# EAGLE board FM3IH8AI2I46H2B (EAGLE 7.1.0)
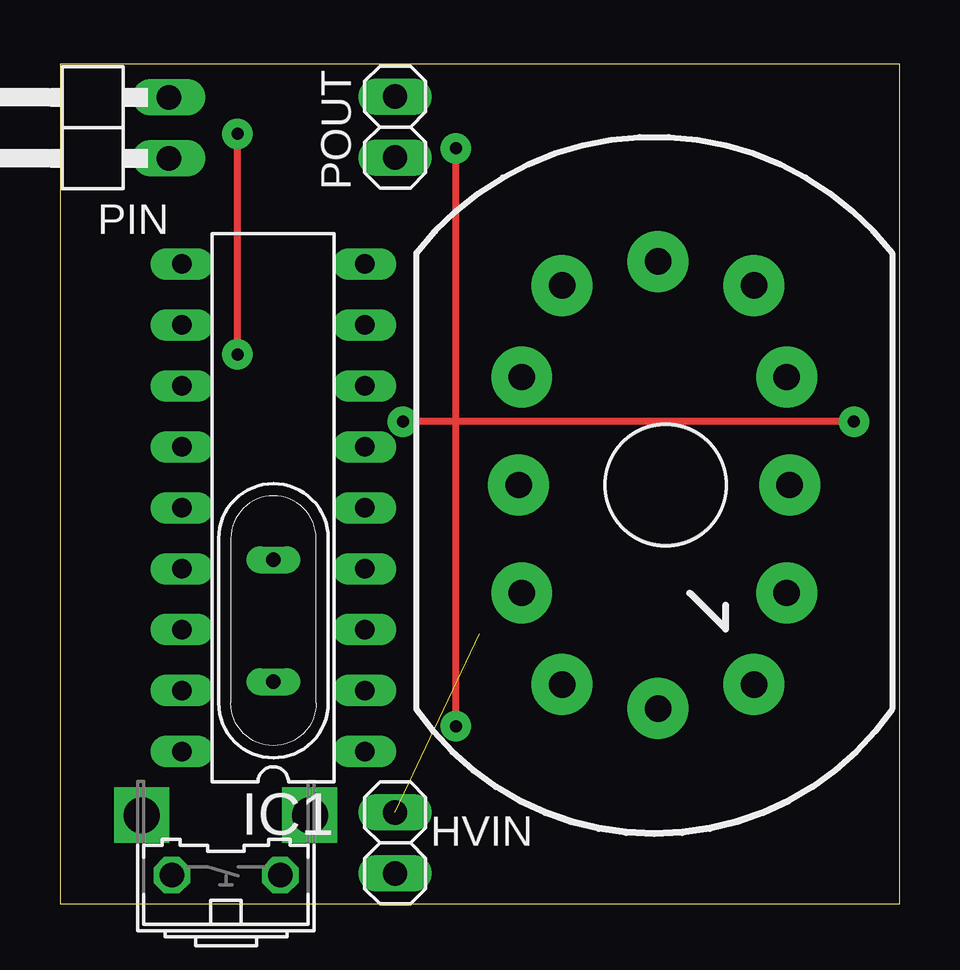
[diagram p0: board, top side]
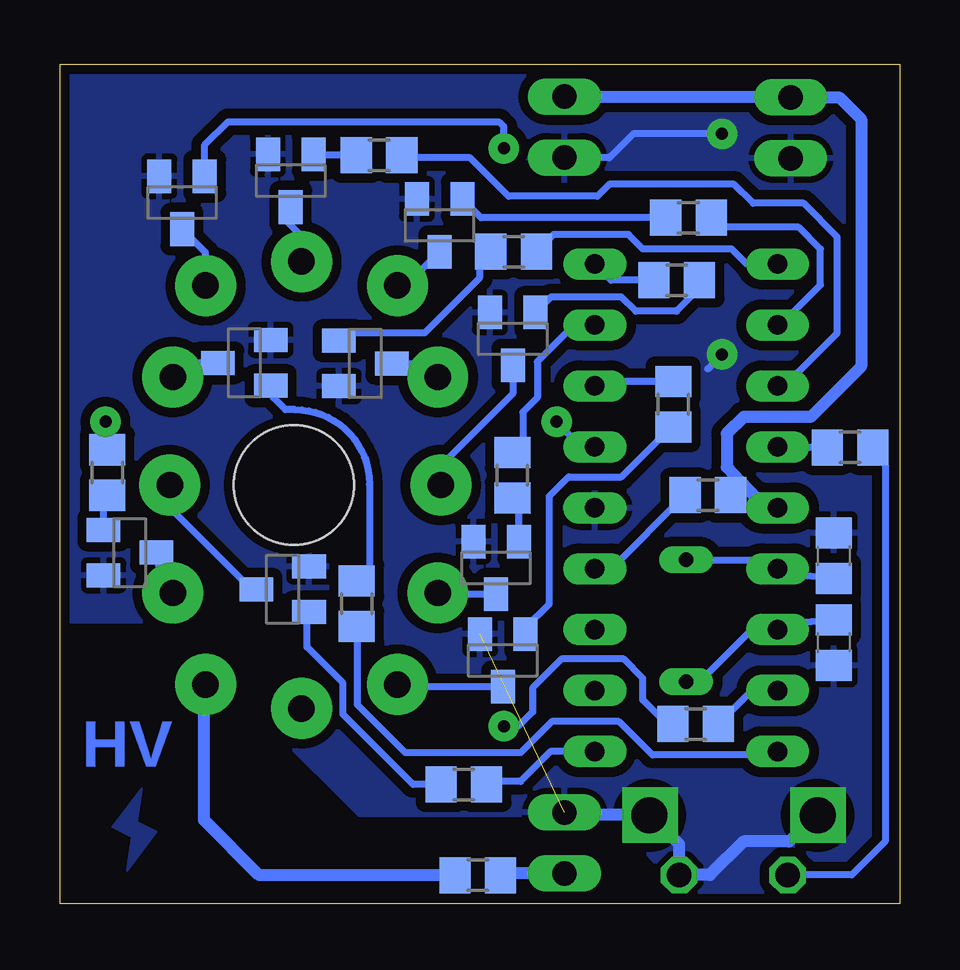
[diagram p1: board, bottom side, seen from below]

Size 35 x 35 mm. Coordinates in mm from the lower left corner, seen from the top.
Outline: 0,0 35,0 35,35 0,35 0,0
Copper layers (1*16): Top 0.035mm / dielectric 1.5mm / Bottom 0.035mm
Design rules "default *": minimum track width 0.2mm, minimum drill 0.4mm, track to track 0.25mm, track to pad 0.2mm, pad to pad 0.2mm, via to via 0.2mm, smd to smd 0.1mm, copper to edge 0.2mm, drill to drill 8mil, minimum pad ring 10mil, minimum via ring 8mil, stop-mask expansion 4mil, vias tented up to drill 0mil, thermal gap 10mil

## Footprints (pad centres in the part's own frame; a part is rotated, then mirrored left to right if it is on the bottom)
C0805 = smd 1.3 x 1.5: 1 -0.95,0; 2 0.95,0
1X02 = drill 1.016 long: 1 -1.27,0; 2 1.27,0
DIL18 = drill 0.813 long: 1 -10.16,-3.81; 2 -7.62,-3.81; 3 -5.08,-3.81; 4 -2.54,-3.81; 5 0,-3.81; 6 2.54,-3.81; 7 5.08,-3.81; 8 7.62,-3.81; 9 10.16,-3.81; 10 10.16,3.81; 11 7.62,3.81; 12 5.08,3.81; 13 2.54,3.81; 14 0,3.81; 15 -2.54,3.81; 16 -5.08,3.81; 17 -7.62,3.81; 18 -10.16,3.81
IN-12 = drill 1.1 pad 2.54: 0 5.048,-4.5; 1 -4.317,-8.318; 2 -6,-4.5; 3 -6.127,0; 4 -6,4.5; 5 -4.317,8.318; 6 -0.318,9.318; 7 3.683,8.318; 8 5.048,4.5; 9 5.175,0; A 3.683,-8.318; LHDP -0.318,-9.318 | hole 5: 0,0
1X02/90 = drill 1.016 long: 1 -1.27,-3.81; 2 1.27,-3.81
QS = drill 0.61 long: 1 -2.54,0; 2 2.54,0
R0805 = smd 1.3 x 1.5: 1 -0.95,0; 2 0.95,0
B3F-31XX = drill 1.016 octagon: 1 -2.261,-1.245; 2 2.261,-1.245 | drill 1.499 pad 2.159: 3 -3.505,1.245; 4 3.505,1.245
SOT23-BEC = smd 1 x 1.4: B -0.95,-1.1; C 0,1.1; E 0.95,-1.1

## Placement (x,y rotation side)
C1  22p  [C0805]  2.74,10.89 90 bottom
C2  22p  [C0805]  2.74,14.51 270 bottom
HVIN  [1X02]  13.97,2.54 270 top
IC1  PIC16F84AP  [DIL18]  8.89,16.51 90 top
N1  IN-12A  [IN-12]  25.25,17.46 0 top
PIN  [1X02/90]  0.73,32.35 90 top
POUT  [1X02]  13.97,32.38 90 top
Q1  [QS]  8.9,11.8 270 top
R1  100k  [R0805]  17.58,1.19 0 bottom
R2  1k  [R0805]  7.99,17.04 180 bottom
R3  470R  [R0805]  2.06,19.03 0 bottom
R5  [R0805]  9.43,20.82 270 bottom
R6  [R0805]  16.14,17.87 270 bottom
R7  [R0805]  9.29,26 0 bottom
R8  [R0805]  16.09,27.18 180 bottom
R9  [R0805]  8.8,28.6 180 bottom
R10  [R0805]  21.7,31.2 180 bottom
R11  [R0805]  8.5,7.5 180 bottom
R12  [R0805]  22.63,12.51 90 bottom
R13  [R0805]  18.16,4.98 180 bottom
R14  [R0805]  33.02,17.98 270 bottom
S1  [B3F-31XX]  6.92,2.44 0 top
T1  [SOT23-BEC]  16.54,10.15 180 bottom
T2  [SOT23-BEC]  16.82,14 180 bottom
T3  [SOT23-BEC]  16.12,23.55 180 bottom
T4  [SOT23-BEC]  22.27,22.53 270 bottom
T5  [SOT23-BEC]  19.18,28.29 180 bottom
T6  [SOT23-BEC]  25.38,30.14 180 bottom
T7  [SOT23-BEC]  29.91,29.23 180 bottom
T8  [SOT23-BEC]  27.32,22.55 90 bottom
T9  [SOT23-BEC]  25.71,13.12 90 bottom
T10  [SOT23-BEC]  32.09,14.64 270 bottom

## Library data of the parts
C1 C2 R1-R3 R5-R14 = rcl
HVIN PIN POUT = pinhead
IC1 = microchip; MF: MICROCHIP; MPN: PIC16F84A-04I/P; OC_FARNELL: 9760865; OC_NEWARK: 69K7635
N1 = russian-nixies
Q1 = special
S1 = switch-omron; MPN: B3F-3100; OC_FARNELL: 959704; OC_NEWARK: 36M3582
T1-T10 = transistor

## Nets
+5V: IC1.14 PIN.2 POUT.2 R2.1
GND: C1.1 C2.1 HVIN.1 IC1.5 PIN.1 POUT.1 S1.2 T1.E T2.E T3.E T4.E T5.E T6.E T7.E T8.E T9.E T10.E
N$1: N1.0 T10.C
N$2: N1.9 T9.C
N$3: N1.8 T8.C
N$4: N1.7 T7.C
N$5: N1.6 T6.C
N$6: N1.5 T5.C
N$7: N1.1 T1.C
N$8: N1.2 T2.C
N$9: N1.3 T3.C
N$10: N1.4 T4.C
N$11: C1.2 IC1.16 Q1.2
N$12: IC1.4 R2.2
N$13: C2.2 IC1.15 Q1.1
N$14: IC1.13 R3.1
N$15: R3.2 S1.1
N$16: IC1.6 R14.1
N$17: IC1.7 R5.1
N$18: R5.2 T1.B
N$19: R6.2 T2.B
N$20: R7.2 T3.B
N$21: IC1.8 R6.1
N$22: N1.A R1.1
N$23: IC1.9 R7.1
N$24: IC1.10 R8.1
N$25: IC1.11 R9.1
N$26: IC1.12 R10.1
N$27: IC1.17 R11.1
N$28: IC1.18 R12.1
N$29: IC1.1 R13.1
N$32: R8.2 T4.B
N$33: R9.2 T5.B
N$34: R10.2 T6.B
N$35: R11.2 T7.B
N$36: R12.2 T8.B
N$37: R13.2 T9.B
N$38: R14.2 T10.B
V+: HVIN.2 R1.2

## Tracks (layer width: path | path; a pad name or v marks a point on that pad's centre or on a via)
+5V
  Bottom 0.3: IC1.14 5.6,16.51 | R2.1 7.44,16.83 6.65,17.62
  Bottom 0.5: POUT.2 13.94,33.62 PIN.2 2.52,33.62 1.6,32.7 1.6,22.4 3.7,20.3 6.5,20.3 7.2,19.6 7.2,18.21 6.65,17.62 5.6,16.51
GND  (via drill 0.5 pad 1.27, 1 pad 2.3)  (1 unrouted)
  Top 0.3: v7.4,22.9 v7.4,32.1
  Bottom 0.3: 8,22.3 v7.4,22.9 | v7.4,32.1 11.1,32.1 12.1,31.1 13.96,31.1 POUT.1
  Bottom 0.5: v3.4,3.7 3.5,3.7 4.6,2.6 6.5,2.6 7.9,1.2 S1.2 9.18,2.48 v10.4,3.7 13.86,3.7 HVIN.1
  pour Bottom (isolate 0.4): 0.3,0.3 8.7,0.3 12.1,3.7 22.5,3.7 26.1,7.3 26.1,10.1 27.8,11.8 34.7,11.8 34.7,34.7 0.3,34.7
N$1
  Bottom 0.3: T10.C 30.89,14.05 N1.0
N$2
  Bottom 0.3: T9.C 26.82,12.91 30.3,16.4 30.3,17.34 N1.9
N$3
  Bottom 0.3: T8.C 29.7,22.55 N1.8
N$4
  Bottom 0.3: N1.7 28.93,27.15 T7.C
N$5
  Bottom 0.3: N1.6 24.93,27.83 25.6,28.5 25.6,28.82 T6.C
N$6
  Bottom 0.3: N1.5 20.58,25.78 T5.C
N$7
  Bottom 0.3: T1.C 20.84,9.05 N1.1
N$8
  Bottom 0.3: T2.C 19.19,12.9 N1.2
N$9
  Bottom 0.3: T3.C 16.12,21.27 19.1,18.3 19.1,17.48 N1.3
N$10
  Bottom 0.3: T4.C 19.82,22.53 N1.4
N$11
  Bottom 0.3: C1.2 4.87,11.64 IC1.16 5.11,11.4 6.2,11.4 8.34,9.26 Q1.2
N$12
  Bottom 0.3: IC1.4 12.01,13.97 R2.2
N$13
  Bottom 0.3: C2.2 4.87,13.76 IC1.15 5.45,14.34 Q1.1
N$14
  Bottom 0.3: R3.1 5.06,19.03 IC1.13
N$15
  Bottom 0.3: R3.2 1.11,18.81 0.6,18.3 0.6,2.6 2,1.2 S1.1
N$16  (via drill 0.5 pad 1.27)
  Top 0.3: v33.1,20.1 v14.3,20.1
  Bottom 0.3: v14.3,20.1 13.25,19 IC1.6 | v33.1,20.1 33.1,19.61 R14.1
N$17
  Bottom 0.3: R5.1 12.38,21.77 IC1.7
N$18
  Bottom 0.3: T1.B 15.59,11.51 14.6,12.5 14.6,17 13.8,17.8 11.6,17.8 10.1,19.3 9.4,19.9 R5.2
N$19
  Bottom 0.3: T2.B 15.87,17.25 R6.2
N$20
  Bottom 0.3: R7.2 8.34,25.66 9.3,24.7 11,24.7 11.6,25.3 14.53,25.3 T3.B
N$21
  Bottom 0.3: IC1.8 13.57,24.13 15.1,22.6 15.1,21.1 15.7,20.5 15.7,19.26 R6.1
N$22
  Bottom 0.5: R1.1 26.69,1.19 29,3.5 29,9.11 N1.A
N$23
  Bottom 0.3: R7.1 12.03,26 IC1.9
N$24
  Bottom 0.3: IC1.10 6.37,26.67 7,27.3 10.7,27.3 11.3,27.9 14.42,27.9 R8.1
N$25
  Bottom 0.3: IC1.11 4.97,24.13 3.3,25.8 3.3,27.3 4.2,28.2 7.45,28.2 R9.1
N$26
  Bottom 0.3: IC1.12 4.81,21.59 2.6,23.8 2.6,27.8 4,29.2 6.1,29.2 6.9,30 12.1,30 12.6,29.5 16.3,29.5 17.9,31.1 20.65,31.1 R10.1
N$27
  Bottom 0.3: IC1.17 6.16,8.89 R11.1
N$28
  Bottom 0.3: IC1.18 6.05,6.35 6.2,6.2 10.3,6.2 11.7,7.6 14.5,7.6 15.8,6.3 20.6,6.3 22.6,8.3 22.6,11.39 R12.1
N$29
  Bottom 0.3: IC1.1 14.55,6.35 15.8,5.1 17.09,5.1 R13.1
N$30
  pour Bottom: 31.6,4.8 31.8,3.4 31,3 32.2,1.4 32,2.8 32.8,3.2
N$32
  Bottom 0.3: R8.2 17.52,26.58 17.52,26.08 19.8,23.8 23.05,23.8 T4.B
N$33
  Bottom 0.3: R9.2 17.44,28.6 T5.B
N$34
  Bottom 0.3: R10.2 24.38,31.2 T6.B
N$35  (via drill 0.5 pad 1.27)
  Top 0.3: v16.5,7.4 v16.5,31.5
  Bottom 0.3: R11.2 9.7,7.5 10.7,8.5 10.7,9.4 11.5,10.2 14.1,10.2 15.3,9 15.3,8 15.9,7.4 v16.5,7.4 | v16.5,31.5 16.5,32.4 16.7,32.6 28,32.6 28.96,31.64 T7.B
N$36
  Bottom 0.3: R12.2 22.1,13.89 22.1,17.5 arc-90 25.2,20.6 25.6,20.6 26.1,21.1 26.1,21.59 T8.B
N$37
  Bottom 0.3: R13.2 20.28,4.98 23.2,7.9 23.2,9.2 24.7,10.7 24.7,12.08 T9.B
N$38
  Bottom 0.3: T10.B 33.19,16.47 R14.2
V+
  Bottom 0.5: HVIN.2 16.55,1.27 R1.2

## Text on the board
Bottom: HV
